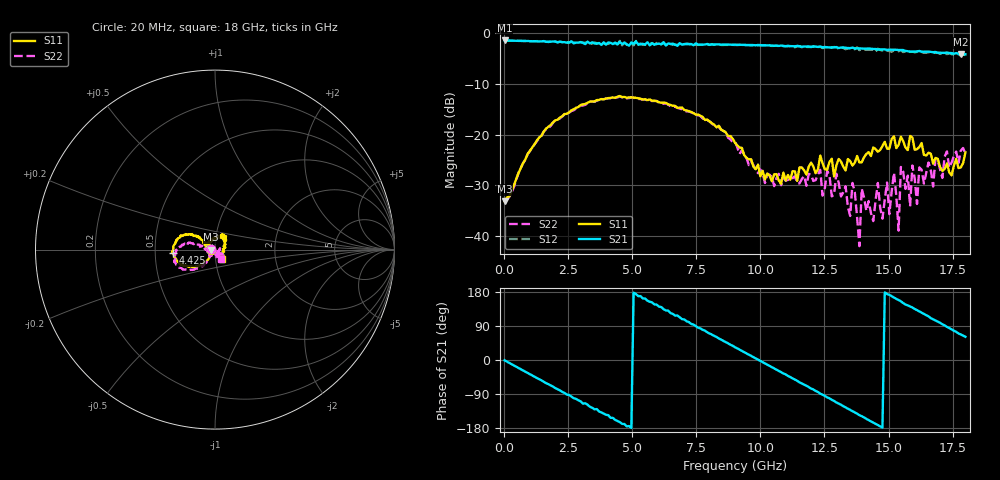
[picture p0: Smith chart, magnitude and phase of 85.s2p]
!Agilent Technologies,N5230A,US43500223,A.07.50.48
!Agilent N5230A: A.07.50.48
!Date: Saturday, January 16, 2016 20:58:16
!Correction: S11(Full 2 Port(1,2))
!S21(Full 2 Port(1,2))
!S12(Full 2 Port(1,2))
!S22(Full 2 Port(1,2))
!S2P File: Measurements: S11, S21, S12, S22:
# Hz S  dB  R 50
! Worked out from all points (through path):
!   201 points, 20 MHz to 18 GHz, reference 50 ohm
!   highest |S21| = -1.42 dB at 20 MHz (marker M1); lowest = -4.2 dB at 17.82 GHz (marker M2)
!   group delay of S21, straight-line fit = 101 ps
!   lowest |S11| = -33.2 dB at 20 MHz (marker M3), VSWR 1.04, Z = 47.9 + j0.0362 ohm
!   |S11| at or under -10 dB: start of sweep to end of sweep
!   |S22| runs from -42.0 to -12.5 dB; largest |S21 - S12| = 0.072
!   S11 on the Smith chart (normalised r, x): 20 MHz: 0.96, +0.00; 4.425 GHz: 0.62, -0.03; 18 GHz: 1.07, -0.12
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2e7  -33.19 179.0  -1.42 -0.8  -1.42 -0.9  -32.75 178.3
1.5483e9  -19.40 -130.9  -1.54 -57.4  -1.54 -57.8  -19.41 -125.5
3.0766e9  -14.04 -154.3  -1.89 -115.2  -1.84 -114.7  -14.25 -144.5
4.4251e9  -12.54 -175.3  -2.17 -160.9  -2.20 -161.0  -12.66 -161.6
6.0433e9  -13.63 161.2  -2.04 140.6  -2.23 137.7  -13.72 179.0
7.4817e9  -16.07 148.4  -1.99 89.6  -2.25 87.0  -16.24 167.0
9.01e9  -21.60 141.3  -2.25 33.8  -2.31 30.9  -21.37 169.3
1.20666e10  -26.29 155.4  -2.61 -77.7  -2.59 -81.8  -29.16 -143.7
1.3505e10  -25.21 122.6  -2.94 -131.4  -2.96 -136.3  -36.07 -117.6
1.35949e10  -26.12 118.1  -2.82 -135.1  -3.16 -140.0  -29.55 -127.8
1.38646e10  -25.53 105.1  -2.98 -145.4  -3.33 -150.0  -42.03 -96.8
1.39545e10  -25.46 104.6  -3.00 -148.2  -3.13 -151.2  -30.67 -128.3
1.50333e10  -22.79 74.2  -3.24 171.7  -3.49 166.7  -35.71 -96.1
1.52131e10  -20.34 58.2  -3.22 164.6  -3.37 161.1  -27.52 -46.1
1.53929e10  -22.04 64.3  -3.30 158.0  -3.53 155.4  -38.96 -49.0
1.54828e10  -20.41 64.7  -3.30 155.0  -3.33 150.2  -26.40 -29.7
1.58424e10  -20.27 50.6  -3.62 141.2  -3.67 138.5  -34.17 -42.5
1.59323e10  -20.60 50.3  -3.61 138.5  -3.64 134.6  -26.11 -40.0
1.61121e10  -22.88 43.0  -3.59 131.5  -3.65 126.6  -33.70 -15.1
1.6202e10  -22.46 43.3  -3.49 128.2  -3.83 123.6  -26.48 -33.4
1.78202e10  -26.50 -58.4  -4.17 67.5  -4.43 62.3  -23.16 -42.4
1.8e10  -23.53 -55.5  -4.14 61.2  -4.30 54.8  -23.81 -58.6
